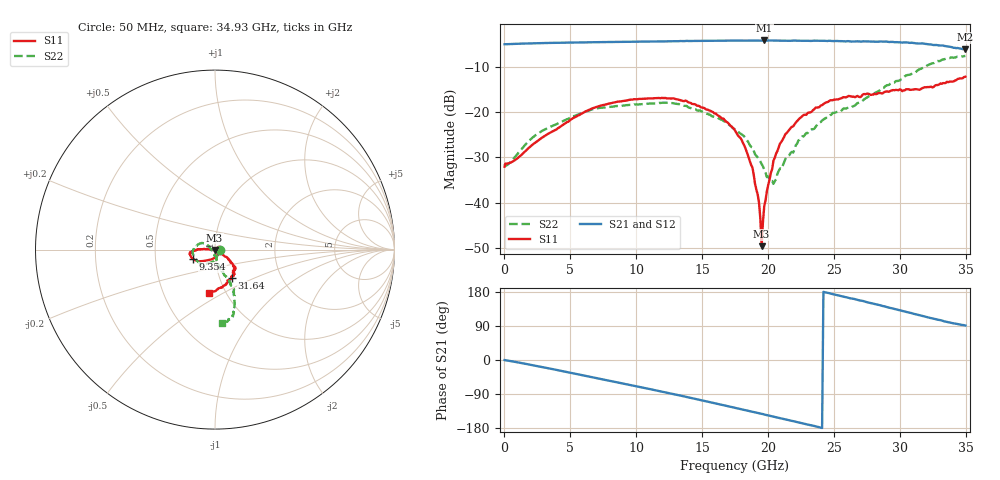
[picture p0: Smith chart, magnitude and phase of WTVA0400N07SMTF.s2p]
! 50 ohm 2-Port S-parameters measured by Modelithics Inc support@modelithics.com  Tampa, FL USA 813-866-6335 (February 2024)
! Smiths Interconnect,  4dB P/N: WTVA0400N07SMTF, Temperature: 0 C
! Board: 10 mil Rogers 4350B, Mounting Pad Dimensions: Length: 15 mils, Width: 25 mils, Gap: 40 mils.
# Hz S RI R 50
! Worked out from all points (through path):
!   352 points, 50 MHz to 34.93 GHz, reference 50 ohm
!   highest |S21| = -4.26 dB at 19.7 GHz (marker M1); lowest = -6.2 dB at 34.93 GHz (marker M2)
!   group delay of S21, straight-line fit = 21.7 ps
!   lowest |S11| = -49.6 dB at 19.5 GHz (marker M3), VSWR 1.01, Z = 49.8 - j0.252 ohm
!   |S11| at or under -10 dB: start of sweep to end of sweep
!   |S22| runs from -35.8 to -7.7 dB; largest |S21 - S12| = 0.0039
!   S11 on the Smith chart (normalised r, x): 50 MHz: 1.05, -0.00; 9.354 GHz: 0.78, -0.08; 31.64 GHz: 1.14, -0.37; 34.93 GHz: 0.83, -0.43
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5e7  0.0249 -0.00125  0.556 -0.00203  0.5556 -0.00215  0.0266 -0.00129
2.6875e9  -0.00795 -0.049  0.546 -0.1692  0.5456 -0.1692  -0.00258 -0.0593
5.8715e9  -0.0709 -0.0642  0.4498 -0.3706  0.4494 -0.3706  -0.0536 -0.0806
9.354e9  -0.1241 -0.0511  0.2555 -0.5338  0.2547 -0.5337  -0.1026 -0.0598
1.1742e10  -0.14 -0.0261  0.0837 -0.5912  0.0827 -0.5911  -0.1232 -0.0251
1.5125e10  -0.1109 -0.0045  -0.184 -0.5772  -0.1846 -0.5768  -0.0955 0.0285
1.7513e10  -0.0614 0.00339  -0.3617 -0.4914  -0.3623 -0.4907  -0.0562 0.0316
1.82095e10  -0.0421 0.00288  -0.4058 -0.4533  -0.4063 -0.4526  -0.0457 0.0272
1.88065e10  -0.0244 5.61e-05  -0.4438 -0.4184  -0.4439 -0.4178  -0.0365 0.0177
1.9304e10  -0.00973 -0.00263  -0.4695 -0.3866  -0.4701 -0.3855  -0.028 0.0107
1.94035e10  -0.006 -0.00306  -0.4746 -0.381  -0.4753 -0.3799  -0.0269 0.00933
1.9503e10  -0.00216 -0.00253  -0.4798 -0.3753  -0.4799 -0.3747  -0.0256 0.00729
1.9702e10  0.0045 -0.00802  -0.4937 -0.3618  -0.4935 -0.3617  -0.0231 0.00305
2.03985e10  0.0241 -0.0162  -0.5268 -0.31  -0.527 -0.3092  -0.0123 -0.0104
2.0896e10  0.037 -0.0253  -0.546 -0.2701  -0.546 -0.2695  -0.0084 -0.0223
2.1891e10  0.0572 -0.0394  -0.5757 -0.1962  -0.5757 -0.1956  0.00127 -0.0357
2.2289e10  0.0683 -0.0461  -0.586 -0.1611  -0.5863 -0.1597  0.00578 -0.0484
2.33835e10  0.0841 -0.0617  -0.6034 -0.0714  -0.6033 -0.0708  0.0105 -0.0637
2.5672e10  0.1098 -0.0952  -0.5856 0.1314  -0.5853 0.1317  0.0251 -0.1054
2.91545e10  0.103 -0.1307  -0.4376 0.393  -0.4365 0.3938  0.0808 -0.1819
3.1642e10  0.0935 -0.1565  -0.2565 0.507  -0.2557 0.507  0.1076 -0.2828
3.49255e10  -0.034 -0.242  -0.0089 0.4881  -0.00613 0.4879  0.0398 -0.4107
